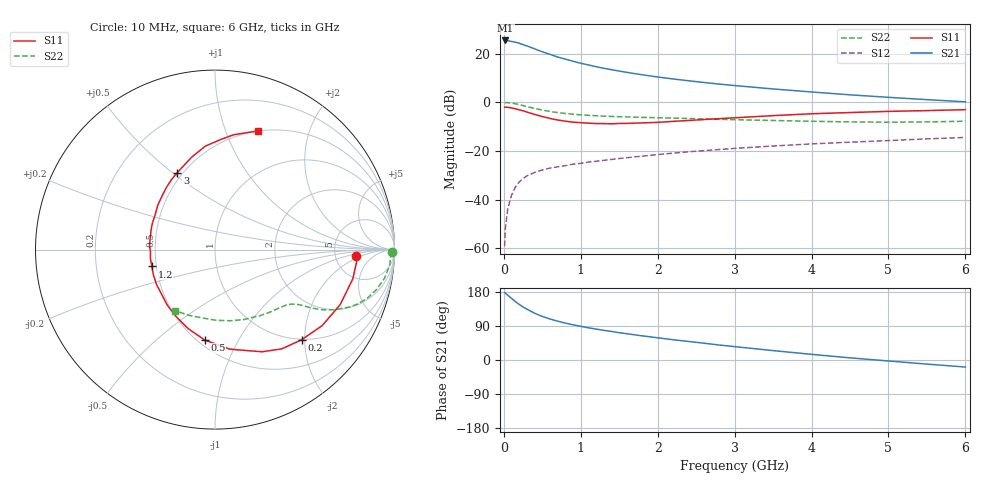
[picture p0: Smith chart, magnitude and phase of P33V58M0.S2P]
! SIEMENS Small Signal Semiconductors
! BFP181
! Si NPN RF Bipolar Junction Transistor in SOT143
! VCE = 3.5 V  IC = 8 mA
! Common Emitter S-Parameters:  March  1996
# GHz  S  MA  R  50
!  f  S11  S21  S12  S22
! GHz  MAG  ANG  MAG  ANG  MAG  ANG  MAG  ANG
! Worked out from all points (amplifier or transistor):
!   36 points, 10 MHz to 6 GHz, reference 50 ohm
!   highest |S21| = 25.4 dB at 20 MHz (marker M1)
!   |S21| within 3 dB of that: start of sweep to 362.6 MHz
!   unconditionally stable (mu >= 1): 1.325 GHz to end of sweep
!   at 250 MHz: K = 0.28, MSG = 27.5 dB, |S12| = -31.4 dB
!   at 1.4 GHz: K = 1.02, MAG = 17.5 dB, |S12| = -23.5 dB
!   at 6 GHz: K = 1.02, MAG = 6.5 dB, |S12| = -14.5 dB
!   S11 on the Smith chart (normalised r, x): 10 MHz: 8.13, -1.53; 200 MHz: 0.99, -1.93; 500 MHz: 0.54, -0.73; 1.2 GHz: 0.47, -0.10; 3 GHz: 0.47, +0.52; 6 GHz: 0.50, +1.30
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0.01  0.7877 -2.6  18.5 177.9  0.0011 77.9  0.9844 -0.8
0.02  0.7917 -5.0  18.57 176.6  0.0026 82.9  0.98 -1.9
0.05  0.7849 -12.0  18.37 171.0  0.0063 85.3  0.9777 -4.9
0.1  0.7617 -23.8  17.73 162.6  0.0123 75.9  0.9582 -9.6
0.15  0.7318 -35.4  17.13 154.2  0.0181 72.0  0.9268 -13.9
0.2  0.6963 -46.2  16.28 146.7  0.0231 67.2  0.8917 -17.6
0.25  0.6664 -56.1  15.24 139.8  0.0268 64.3  0.852 -20.8
0.3  0.6266 -65.3  14.34 134.2  0.0306 60.1  0.8136 -23.2
0.4  0.5609 -81.5  12.49 123.4  0.036 55.7  0.7443 -26.8
0.5  0.5071 -96.5  10.85 115.0  0.0406 51.2  0.6897 -29.1
0.6  0.464 -109.1  9.621 108.2  0.0443 49.8  0.6454 -30.6
0.7  0.4305 -120.4  8.472 102.4  0.047 48.3  0.6114 -31.6
0.9  0.3887 -139.4  6.944 93.0  0.0534 47.1  0.5663 -33.0
1.1  0.3712 -157.6  5.827 84.9  0.0588 46.2  0.5374 -34.4
1.2  0.364 -165.1  5.368 81.6  0.0612 45.7  0.5273 -35.2
1.7  0.371 164.2  3.865 66.5  0.0752 45.5  0.493 -40.0
2.2  0.4037 142.2  3.004 53.5  0.0897 43.6  0.4707 -46.2
3  0.4779 116.0  2.2 35.3  0.1124 39.3  0.4371 -58.5
3.5  0.53 104.4  1.871 24.8  0.1259 36.2  0.4214 -67.7
4.5  0.6134 87.2  1.418 5.7  0.1508 28.7  0.394 -89.0
5.5  0.672 75.4  1.128 -10.8  0.1764 22.1  0.3939 -111.6
6  0.7029 70.1  1.019 -18.6  0.1888 18.1  0.4065 -123.1
